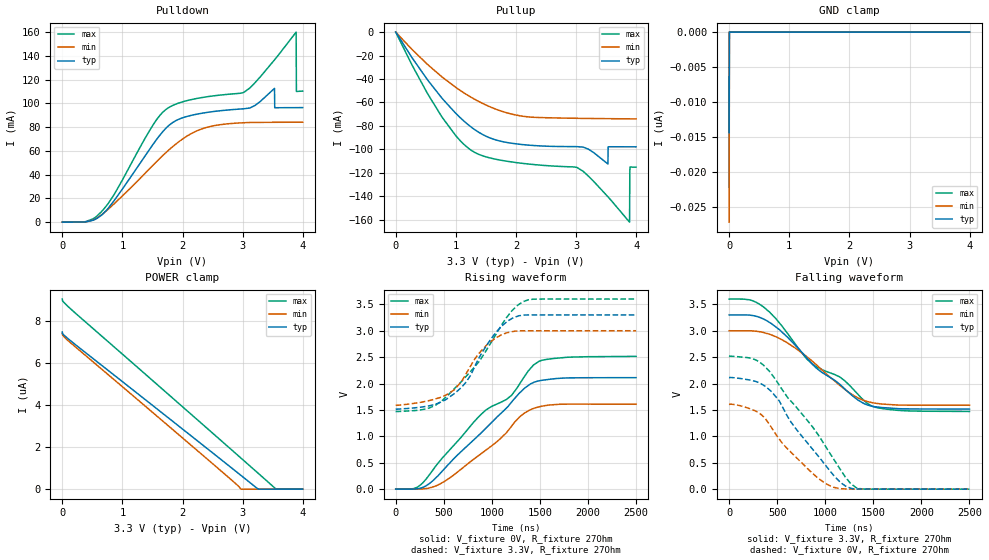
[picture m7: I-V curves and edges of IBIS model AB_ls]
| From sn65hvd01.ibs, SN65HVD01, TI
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|   Model
[Model]   AB_ls
Model_type   I/O
Polarity   Non-Inverting
Enable   Active-Low
Vinl = 0.99
Vinh = 2.31
Vmeas = 1.65
Vref = 1.65
Cref = 1pF
Rref = 27
|   typ   min   max
C_comp   2.359pF   1.818pF   2.464pF
[Voltage Range]   3.3   3   3.6
[Temperature Range]   27   125   -40
[Pullup Reference]   3.3   3   3.6
[Pulldown Reference]   -0   -0   -0
[Power Clamp Reference]   3.3   3   3.6
[GND Clamp Reference]   -0   -0   -0
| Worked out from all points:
|   slope of the pulldown table from 0 to 0.495 V, typ, clamps not added: 340 ohm
|   slope of the pullup table from 0 to 0.495 V, typ, clamps not added: 12.9 ohm
|   falling waveform, V_fixture 3.3V, R_fixture 27Ohm: 20-80 % time 649ns typ, 566ns min, 777ns max; typ from 3.3 V to 1.52 V
|   rising waveform, V_fixture 0V, R_fixture 27Ohm: 20-80 % time 698ns typ, 605ns min, 850ns max; typ from 0 V to 2.11 V
|   rising waveform, V_fixture 3.3V, R_fixture 27Ohm: 20-80 % time 381ns typ, 340ns min, 519ns max; typ from 1.52 V to 3.3 V
|   falling waveform, V_fixture 0V, R_fixture 27Ohm: 20-80 % time 503ns typ, 457ns min, 604ns max; typ from 2.11 V to 0 V
[Pulldown]
|   Voltage   I(typ)   I(min)   I(max)
0V        -1.28nA    3.402nA    -6.697nA
396mV     302.7uA    326.3uA    558.1uA
648mV     5.731mA    6.042mA    8.677mA
1.56V     69.14mA    50.66mA    85.8mA
1.912V    86.16mA    66.79mA    99.93mA
2.344V    91.97mA    79.01mA    105.2mA
3.016V    95.52mA    83.76mA    109.3mA
3.528V    112.7mA    84.16mA    136.7mA
3.532V    96.38mA    84.16mA    137mA
3.888V    96.5mA     84.22mA    160.1mA
3.892V    96.5mA     84.22mA    110.1mA
3.996V    96.51mA    84.23mA    110.4mA
[GND Clamp]
|   Voltage   I(typ)   I(min)   I(max)
0V        -14.37nA   -27.11nA   -22.07nA
4mV       0A         0A         0A
8mV       0A         0A         0A
3.996V    0A         0A         0A
[Pullup]
|   Voltage   I(typ)   I(min)   I(max)
0V        -602.5nA   -398.4nA   -925.3nA
760mV     -55.79mA   -37.81mA   -71.68mA
1.056V    -72.2mA    -49.18mA   -91.7mA
1.32V     -83.42mA   -57.52mA   -102.8mA
2.064V    -95.7mA    -71.37mA   -111.7mA
3.016V    -97.72mA   -73.54mA   -115.5mA
3.528V    -112.5mA   -73.85mA   -140.5mA
3.532V    -97.85mA   -73.85mA   -140.7mA
3.888V    -97.85mA   -74mA      -162.2mA
3.892V    -97.85mA   -74.01mA   -118.6mA
3.896V    -97.85mA   -74.01mA   -115.1mA
3.996V    -97.86mA   -74.05mA   -115.2mA
[POWER Clamp]
|   Voltage   I(typ)   I(min)   I(max)
0V        7.47uA     7.414uA    9.032uA
4mV       7.384uA    7.323uA    8.944uA
116mV     7.102uA    7.007uA    8.625uA
2.512V    1.696uA    1.179uA    2.629uA
2.88V     860.4nA    269.2nA    1.704uA
2.972V    651nA      0A         1.473uA
3.256V    417.8pA    0A         757.1nA
3.556V    0A         0A         0A
3.996V    0A         0A         0A
[Ramp]
R_load = 27
|   typ   min   max
dV/dt_r   1.26709/6.98324e-07   0.964755/6.05176e-07   1.50874/8.49959e-07
dV/dt_f   1.07006/6.4907e-07   0.845631/5.66349e-07   1.27693/7.77309e-07
[Falling Waveform]
V_fixture = 3.3V
V_fixture_min = 3V
V_fixture_max = 3.6V
R_fixture = 27Ohm
C_fixture = 0F
|   Time   V(typ)   V(min)   V(max)
0s        3.3V       3V         3.6V
245.7ns   3.287V     2.996V     3.567V
442.7ns   3.132V     2.919V     3.311V
806.1ns   2.49V      2.511V     2.467V
901.7ns   2.302V     2.365V     2.328V
1.15us    1.986V     1.967V     2.126V
1.239us   1.839V     1.84V      1.99V
1.49us    1.569V     1.637V     1.569V
1.82us    1.521V     1.591V     1.485V
2.5us     1.516V     1.591V     1.472V
[Rising Waveform]
V_fixture = 0V
V_fixture_min = 0V
V_fixture_max = 0V
R_fixture = 27Ohm
C_fixture = 0F
|   Time   V(typ)   V(min)   V(max)
0s        4.465uV    3.796uV    6.805uV
231.4ns   9.163mV    1.104mV    45.15mV
353ns     109.5mV    24.41mV    278.1mV
494.3ns   362mV      132.7mV    609.2mV
935.4ns   1.15V      735.2mV    1.496V
1.207us   1.654V     1.198V     1.781V
1.34us    1.912V     1.442V     2.136V
1.49us    2.052V     1.56V      2.421V
1.784us   2.106V     1.61V      2.497V
2.5us     2.112V     1.608V     2.515V
[Rising Waveform]
V_fixture = 3.3V
V_fixture_min = 3V
V_fixture_max = 3.6V
R_fixture = 27Ohm
C_fixture = 0F
|   Time   V(typ)   V(min)   V(max)
0s        1.516V     1.591V     1.471V
310.6ns   1.566V     1.663V     1.518V
482.9ns   1.663V     1.751V     1.678V
606.7ns   1.807V     1.879V     1.898V
727.1ns   2.015V     2.17V      2.126V
858.4ns   2.457V     2.554V     2.398V
1us       2.867V     2.811V     2.803V
1.163us   3.183V     2.964V     3.275V
1.32us    3.293V     2.999V     3.547V
2.5us     3.3V       3V         3.6V
[Falling Waveform]
|Gnd
V_fixture = 0V
V_fixture_min = 0V
V_fixture_max = 0V
R_fixture = 27Ohm
C_fixture = 0F
|   Time   V(typ)   V(min)   V(max)
0s        2.112V     1.607V     2.516V
280.2ns   2.037V     1.474V     2.444V
418.3ns   1.883V     1.229V     2.234V
522.4ns   1.669V     945.6mV    1.967V
606.7ns   1.38V      763.8mV    1.74V
952.8ns   568mV      170.8mV    955.3mV
1.163us   118.5mV    8.59mV     354.4mV
1.264us   20.66mV    1.417mV    106.7mV
1.32us    4.846mV    1.353mV    29.16mV
2.5us     27uV       22.56uV    38.34uV
